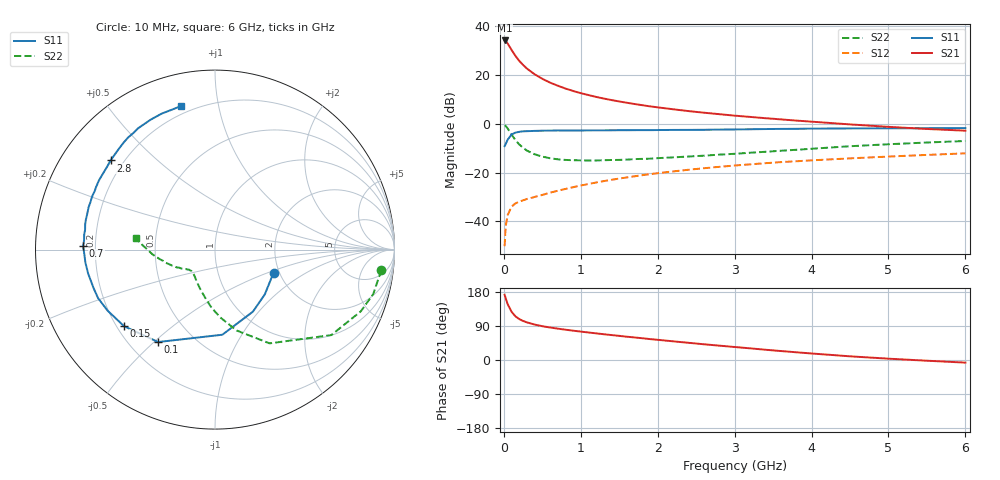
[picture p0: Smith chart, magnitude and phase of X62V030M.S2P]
! SIEMENS Small Signal Semiconductors
! BFP193W
! Si NPN RF Bipolar Junction Transistor in SOT343
! VCE = 2 V  IC = 30 mA
! Common Emitter S-Parameters:  April 1994
# GHz  S  MA  R  50
!  f  S11  S21  S12  S22
! GHz  MAG  ANG  MAG  ANG  MAG  ANG  MAG  ANG
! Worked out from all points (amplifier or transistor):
!   40 points, 10 MHz to 6 GHz, reference 50 ohm
!   highest |S21| = 34.3 dB at 10 MHz (marker M1)
!   |S21| within 3 dB of that: start of sweep to 83.46 MHz
!   unconditionally stable (mu >= 1): 750 MHz to 3.998 GHz
!   at 200 MHz: K = 0.46, MSG = 28.9 dB, |S12| = -31.9 dB
!   at 1.5 GHz: K = 1.13, MAG = 13.6 dB, |S12| = -22.4 dB
!   at 6 GHz: K = 0.93, MSG = 4.6 dB, |S12| = -12.1 dB
!   lowest NFmin = 1.90 dB at 450 MHz
!   S11 on the Smith chart (normalised r, x): 10 MHz: 1.87, -0.55; 100 MHz: 0.32, -0.52; 150 MHz: 0.23, -0.35; 700 MHz: 0.15, +0.01; 2.8 GHz: 0.15, +0.36; 6 GHz: 0.16, +0.78
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0.01  0.3509 -21.5  51.59 172.1  0.0031 82.9  0.934 -7.0
0.02  0.3733 -42.0  50.75 165.9  0.0062 75.6  0.9156 -15.7
0.03  0.4052 -58.6  49.18 159.3  0.009 72.8  0.8825 -22.9
0.05  0.4761 -85.1  44.56 147.4  0.0135 63.9  0.8043 -36.3
0.1  0.6046 -121.6  33.11 127.4  0.0201 49.1  0.6045 -59.8
0.15  0.6625 -139.9  24.99 115.4  0.0233 42.7  0.4667 -75.0
0.2  0.6883 -150.4  19.69 108.1  0.0255 41.3  0.3795 -85.5
0.25  0.7053 -157.4  16.23 103.0  0.027 41.3  0.3249 -93.3
0.3  0.7095 -162.2  13.67 99.3  0.0288 42.4  0.2835 -99.8
0.4  0.7193 -169.3  10.43 93.5  0.0317 44.5  0.2386 -109.5
0.5  0.7256 -174.2  8.428 89.2  0.0349 47.7  0.2133 -116.8
0.6  0.7287 -178.1  7.046 85.8  0.0388 50.0  0.1976 -122.6
0.7  0.7347 178.6  6.094 82.8  0.0425 52.1  0.1879 -126.8
0.9  0.7335 173.5  4.748 77.4  0.0503 55.1  0.18 -132.9
1.1  0.7369 169.0  3.909 72.6  0.0585 56.9  0.1773 -137.1
1.6  0.7425 159.3  2.715 61.4  0.08 58.3  0.1851 -142.9
2.2  0.7529 149.2  1.999 49.3  0.106 56.6  0.2056 -149.0
2.8  0.7651 139.5  1.585 37.9  0.1317 53.4  0.2343 -154.8
3.2  0.7769 133.3  1.393 30.8  0.1479 50.6  0.256 -159.7
4.5  0.8079 116.3  0.977 9.7  0.1965 41.5  0.3484 -175.5
5.5  0.8153 107.5  0.788 -1.9  0.2312 34.9  0.4154 175.3
6  0.8215 103.5  0.726 -6.9  0.2493 31.9  0.4465 171.8
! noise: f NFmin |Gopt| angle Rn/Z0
0.45  1.9  0.4  180  0.09
0.9  1.95  0.43  -173  0.11
1.8  2.4  0.58  -144  0.24
